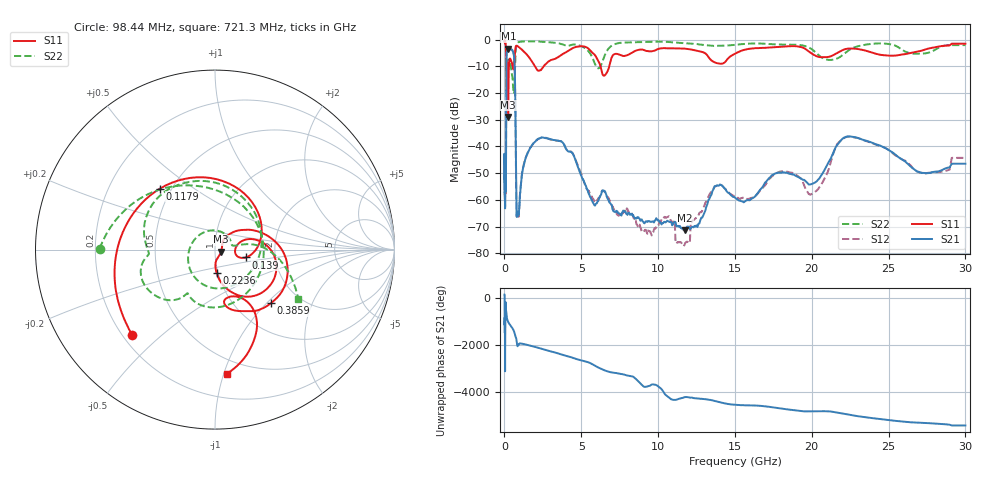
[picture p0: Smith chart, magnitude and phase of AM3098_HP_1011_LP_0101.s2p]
! Date/Time: Thu, Feb 28, 2019 8:43 AM
! Network Analyzer: Agilent Technologies E8364B Rev: A.07.50.67
! Sweep from 0.010 to 30.000 GHz, 1601 Points, Sweep Type: LOG
! Power Supply: 5.023 V, 0.002 A
# Hz S DB R 50
!freq MagS11 AngS11 MagS21 AngS21 MagS12 AngS12 MagS22 AngS22
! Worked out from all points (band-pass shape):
!   1601 points, 10 MHz to 30 GHz, reference 50 ohm
!   highest |S21| = -3.44 dB at 259.9 MHz (marker M1); lowest = -71.3 dB at 11.77 GHz (marker M2)
!   |S21| within 3 dB of the highest: 136.6 MHz to 624 MHz (487.4 MHz wide, 128 % of centre)
!   lowest |S11| = -28.9 dB at 239.9 MHz (marker M3), VSWR 1.07, Z = 53.5 - j1.2 ohm
!   |S11| at or under -10 dB: 200.6 MHz to 291.4 MHz (90.8 MHz wide, 36.9 % of centre); 1.975 GHz to 2.552 GHz (576.7 MHz wide, 25.5 % of centre); 6.252 GHz to 6.824 GHz (571.8 MHz wide, 8.75 % of centre)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
!   |S22| runs from -20.3 to -0.5 dB; largest |S21 - S12| = 0.0091
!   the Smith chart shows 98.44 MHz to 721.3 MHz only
!   S11 on the Smith chart (normalised r, x): 98.44 MHz: 0.24, -0.40; 117.9 MHz: 0.43, +0.37; 139 MHz: 1.41, -0.13; 223.6 MHz: 0.98, -0.26; 385.9 MHz: 1.44, -1.06; 721.3 MHz: 0.39, -1.03
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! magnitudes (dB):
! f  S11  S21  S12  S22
! 10 MHz  -0.3  -42.8  -44.8  -0.5
! 38.04 MHz  -0.4  -61.8  -60.1  -0.8
! 98.44 MHz  -3.6  -53.8  -53.0  -3.8
! 117.9 MHz  -6.8  -20.6  -20.7  -10.8
! 139 MHz  -15.0  -5.9  -5.9  -10.6
! 144.7 MHz  -18.4  -5.2  -5.1  -10.8
! 223.6 MHz  -17.7  -3.5  -3.5  -8.4
! 239.9 MHz  -28.9  -3.4  -3.4  -8.7
! 259.9 MHz  -16.6  -3.4  -3.4  -8.4
! 385.9 MHz  -7.3  -3.7  -3.6  -8.8
! 550.5 MHz  -10.6  -4.4  -4.4  -16.7
! 659.1 MHz  -6.8  -9.6  -9.6  -15.6
! 721.3 MHz  -3.2  -30.9  -30.8  -5.3
! 817.4 MHz  -2.3  -64.9  -65.1  -1.6
! 2.084 GHz  -11.0  -37.6  -37.7  -0.7
! 3.742 GHz  -5.6  -38.3  -38.2  -1.7
! 7.926 GHz  -6.0  -65.2  -64.1  -1.1
! 11.77 GHz  -3.4  -71.3  -76.1  -1.4
! 13.81 GHz  -8.8  -54.6  -54.6  -2.3
! 20.2 GHz  -5.9  -53.5  -57.0  -4.5
! 22.44 GHz  -3.4  -36.2  -36.3  -3.9
! 30 GHz  -1.5  -46.4  -44.3  -2.1
